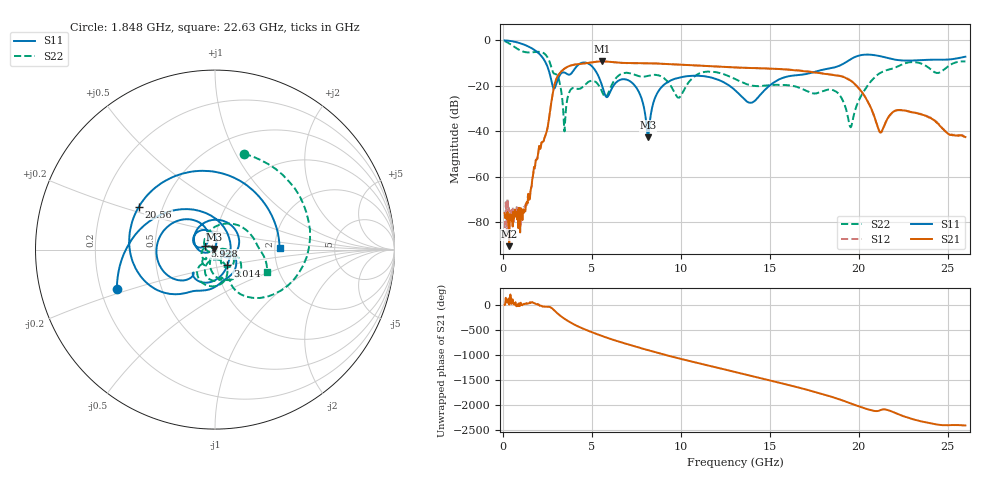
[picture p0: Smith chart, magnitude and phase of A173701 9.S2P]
!  2-Port S-parameters saved by WinCal
! VAR MeasName=S-Parameters (CALIBRATED_DATA) read from VNA (N5245A)
! VAR MeasDate=2017-6-7 10:29:01
! VAR NAME=A173701 9
! VAR FILENAME=A173701 9.S2P
! VAR DATE=2017-6-7 10:29:01
! VAR PHYS_PORTS=1,2
# Hz S DB R 50
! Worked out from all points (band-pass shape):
!   801 points, 100 MHz to 26 GHz, reference 50 ohm
!   highest |S21| = -9.22 dB at 5.571 GHz (marker M1); lowest = -90.7 dB at 359 MHz (marker M2)
!   |S21| within 3 dB of the highest: 3.506 GHz to 14.22 GHz (10.72 GHz wide, 121 % of centre)
!   lowest |S11| = -42.6 dB at 8.161 GHz (marker M3), VSWR 1.01, Z = 49.4 + j0.402 ohm
!   |S11| at or under -10 dB: 2.421 GHz to 4.393 GHz (1.972 GHz wide, 57.9 % of centre); 4.748 GHz to 19.2 GHz (14.45 GHz wide, 121 % of centre)
!   |S22| runs from -40.1 to -0.3 dB; largest |S21 - S12| = 0.0041
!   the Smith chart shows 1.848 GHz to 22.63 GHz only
!   S11 on the Smith chart (normalised r, x): 1.848 GHz: 0.27, -0.18; 3.014 GHz: 1.13, -0.20; 5.928 GHz: 0.89, +0.04; 20.56 GHz: 0.37, +0.23; 22.63 GHz: 2.12, +0.03
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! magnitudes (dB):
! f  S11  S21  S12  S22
! 100 MHz  0.0  -76.1  -87.2  -0.3
! 359 MHz  -0.2  -90.7  -86.3  -1.4
! 1.039 GHz  -1.4  -77.1  -79.1  -4.6
! 1.848 GHz  -4.6  -52.8  -52.7  -5.1
! 3.014 GHz  -19.0  -16.8  -16.8  -15.0
! 3.467 GHz  -14.1  -12.4  -12.4  -40.1
! 4.438 GHz  -9.9  -10.3  -10.3  -20.8
! 5.571 GHz  -19.8  -9.2  -9.2  -22.5
! 5.928 GHz  -24.4  -9.4  -9.4  -23.2
! 7.223 GHz  -18.4  -10.0  -10.0  -14.6
! 8.161 GHz  -42.6  -10.0  -10.1  -15.6
! 8.744 GHz  -22.4  -10.2  -10.2  -15.4
! 9.877 GHz  -16.4  -10.6  -10.7  -25.2
! 13.05 GHz  -21.9  -11.9  -11.9  -17.0
! 17.39 GHz  -14.2  -14.0  -13.9  -23.3
! 18.78 GHz  -11.6  -15.5  -15.3  -22.8
! 19.56 GHz  -8.3  -17.8  -17.7  -38.3
! 20.56 GHz  -6.3  -27.7  -27.7  -19.3
! 21.21 GHz  -6.9  -40.4  -40.6  -14.3
! 21.69 GHz  -7.8  -33.5  -33.7  -12.8
! 22.63 GHz  -8.9  -30.9  -31.0  -10.0
! 26 GHz  -7.2  -42.6  -42.6  -9.3
